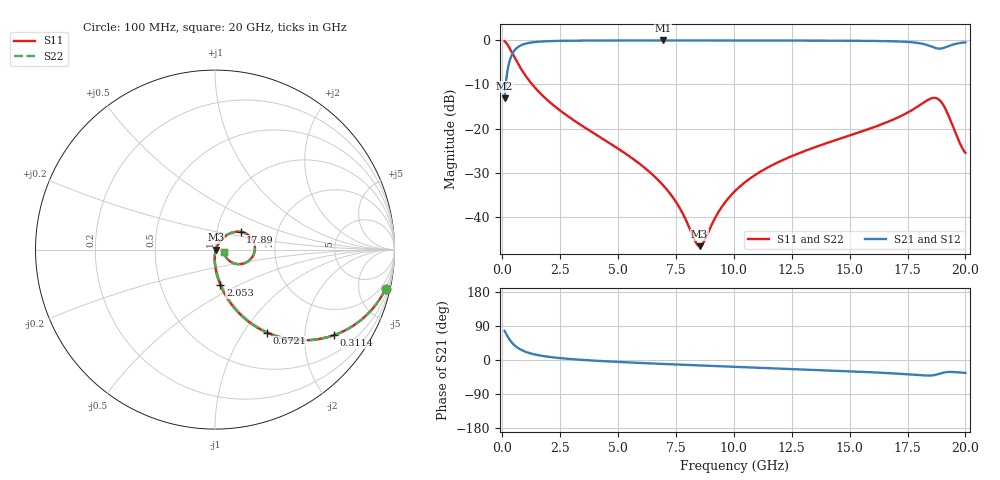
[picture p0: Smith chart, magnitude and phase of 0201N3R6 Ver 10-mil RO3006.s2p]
# GHz S MA R 50
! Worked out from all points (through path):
!   1601 points, 100 MHz to 20 GHz, reference 50 ohm
!   highest |S21| = -0.04 dB at 6.941 GHz (marker M1); lowest = -13.1 dB at 100 MHz (marker M2)
!   group delay of S21, straight-line fit = 8.49 ps
!   lowest |S11| = -46.7 dB at 8.52 GHz (marker M3), VSWR 1.01, Z = 50.4 - j0.131 ohm
!   |S11| at or under -10 dB: 1.292 GHz to end of sweep
!   |S22| runs from -46.7 to -0.2 dB; largest |S21 - S12| = 0
!   S11 on the Smith chart (normalised r, x): 100 MHz: 0.98, -8.71; 311.4 MHz: 0.98, -2.79; 672.1 MHz: 0.98, -1.29; 2.053 GHz: 0.98, -0.40; 17.89 GHz: 1.30, +0.27; 20 GHz: 1.11, -0.04
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0.1  0.9752 -12.9  0.2212 77.0  0.2212 77.0  0.9752 -12.9
0.3114375  0.8161 -35.8  0.5771 54.2  0.5771 54.2  0.8161 -35.8
0.672125  0.5458 -57.9  0.8367 31.9  0.8367 31.9  0.5458 -57.9
1.169625  0.3469 -71.4  0.9363 18.3  0.9363 18.3  0.3469 -71.4
2.052688  0.1988 -81.4  0.9778 8.0  0.9778 8.0  0.1988 -81.4
3.420812  0.1086 -88.0  0.9911 0.4  0.9911 0.4  0.1086 -88.0
6.741625  0.02596 -90.9  0.9954 -9.9  0.9954 -9.9  0.02596 -90.9
6.940625  0.02287 -90.0  0.9954 -10.4  0.9954 -10.4  0.02287 -90.0
7.599812  0.0134 -83.1  0.9954 -12.1  0.9954 -12.1  0.0134 -83.1
8.333625  0.005271 -43.4  0.9952 -13.9  0.9952 -13.9  0.005271 -43.4
8.520188  0.004648 -16.2  0.9951 -14.3  0.9951 -14.3  0.004648 -16.2
8.70675  0.005223 10.9  0.9951 -14.8  0.9951 -14.8  0.005223 10.9
9.415688  0.01222 49.7  0.9948 -16.5  0.9948 -16.5  0.01222 49.7
10.05  0.01957 56.7  0.9944 -18.0  0.9944 -18.0  0.01957 56.7
11.38081  0.03519 59.6  0.9934 -21.1  0.9934 -21.1  0.03519 59.6
13.37081  0.05969 57.7  0.9911 -25.8  0.9911 -25.8  0.05969 57.7
16.69162  0.1202 47.8  0.9766 -34.7  0.9766 -34.7  0.1202 47.8
17.88563  0.1739 34.7  0.9377 -39.4  0.9377 -39.4  0.1739 34.7
18.53237  0.2198 11.3  0.8492 -40.8  0.8492 -40.8  0.2198 11.3
18.88062  0.2102 -12.3  0.8038 -36.3  0.8038 -36.3  0.2102 -12.3
19.24131  0.1461 -33.3  0.8534 -31.7  0.8534 -31.7  0.1461 -33.3
20  0.05296 -17.4  0.9486 -34.0  0.9486 -34.0  0.05296 -17.4
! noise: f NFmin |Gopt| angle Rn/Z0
0.1  0.0008005  0.9468  0.5532  0.003369
2.301  0.004615  0.8006  4.146  0.004793
4.515  0.007666  0.7689  7.771  0.006724
6.729  0.01039  0.7492  11.41  0.008265
8.943  0.013  0.7361  15.04  0.009677
11.14  0.01565  0.7289  18.62  0.01119
13.36  0.01884  0.7308  22.2  0.01344
15.57  0.02467  0.7577  25.79  0.01959
17.79  0.05465  0.8678  29.49  0.08319
20  0.06357  0.8726  33.15  0.09882
